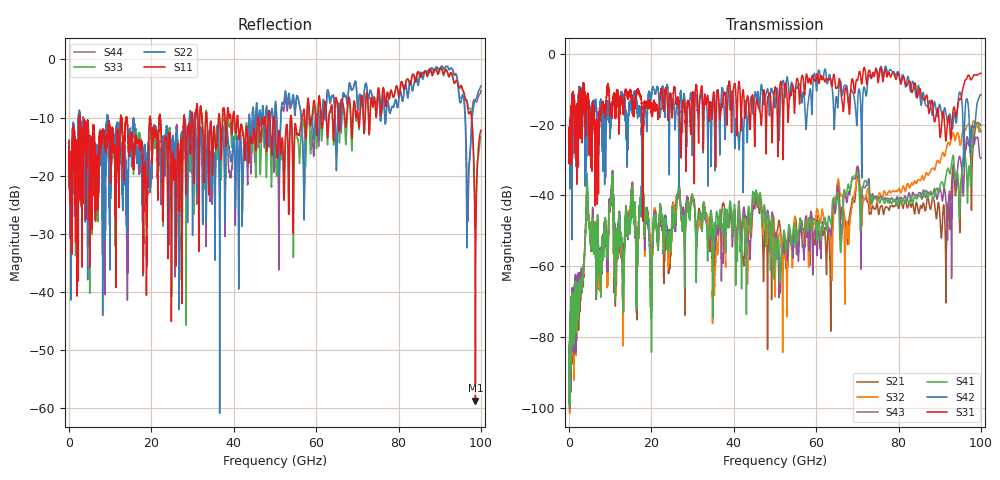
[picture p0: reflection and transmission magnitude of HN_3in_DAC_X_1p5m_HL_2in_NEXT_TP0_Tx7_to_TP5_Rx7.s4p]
# GHz S RI R 45
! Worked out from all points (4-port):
!   4000 points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, 25 MHz to 100 GHz, reference 45 ohm
!   strongest paths, dB at 25 MHz, 25.02 GHz, 50.02 GHz, 75.03 GHz, 100 GHz:
!     S31: -20.8, -18.1, -9.5, -8.0, -5.4
!     S42: -20.8, -16.2, -15.1, -5.7, -11.5
!     S41: -87.4, -45.5, -53.4, -40.6, -21.7
!     S43: -97.5, -46.9, -53.3, -40.9, -29.6
!     S32: -98.9, -47.4, -68.7, -41.0, -21.9
!     S21: -94.9, -46.6, -57.4, -44.1, -20.2
!   lowest |S11| = -58.7 dB at 98.67 GHz (marker M1), VSWR 1.00, Z = 44.9 - j0.0587 ohm
!   |S11| at or under -10 dB: 2.653 GHz to 12.57 GHz (9.914 GHz wide, 130 % of centre); 14.03 GHz to 19.59 GHz (5.561 GHz wide, 33.1 % of centre); 22.16 GHz to 27.84 GHz (5.687 GHz wide, 22.7 % of centre)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
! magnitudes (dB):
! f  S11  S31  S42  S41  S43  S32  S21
! 25 MHz  -14.0  -20.8  -20.8  -87.4  -97.5  -98.9  -94.9
! 10.28 GHz  -13.5  -14.9  -16.3  -39.6  -38.3  -39.2  -40.4
! 51.27 GHz  -14.9  -8.3  -14.3  -64.1  -67.6  -50.6  -49.0
! 69.92 GHz  -9.0  -7.4  -19.6  -33.7  -32.0  -33.7  -35.3
! 91.53 GHz  -1.7  -24.5  -16.8  -34.4  -41.8  -27.3  -70.4
! 98.67 GHz  -58.7  -6.0  -18.7  -19.8  -23.7  -19.8  -20.9
! 100 GHz  -12.2  -5.4  -11.5  -21.7  -29.6  -21.9  -20.2
